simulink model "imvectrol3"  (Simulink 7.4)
settings: Solver=ode23tb  StartTime=0.0  StopTime=1  RelTol=1e-3  AbsTol=1e-3
StartFcn:
  | load('IC3.mat')

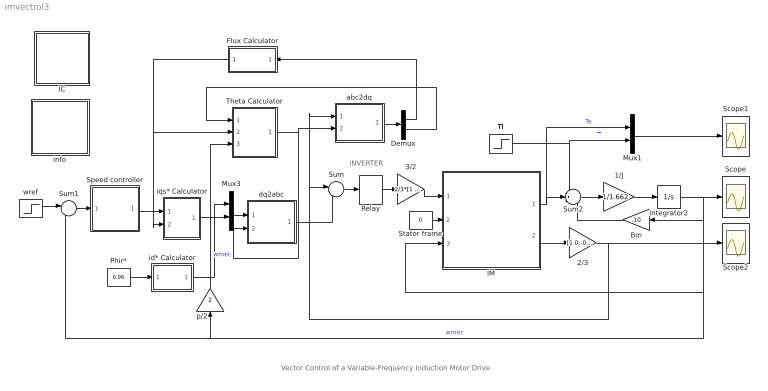
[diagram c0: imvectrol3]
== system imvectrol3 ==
  note: Vector Control of a Variable-Frequency Induction Motor Drive
  note: INVERTER
  1/J : Gain  Gain=1/1.662
  2/3 : Gain  Gain=[1 0;-0.5 sqrt(3)/2;-0.5 -sqrt(3)/2]  Multiplication=Matrix(K*u)
  3/2 : Gain  Gain=2/3*[1 -.5 -.5;0 sqrt(3)/2 -sqrt(3)/2]  Multiplication=Matrix(K*u)
  Bm : Gain  Gain=.10
  Demux : Demux  Outputs=2
  Flux Calculator : Subsystem
  IC : Subsystem
  IM : Subsystem  mask{Rs=0.087, Lsl=0.8e-3, Rr=0.228, Lrl=0.8e-3, Lm=34.7e-3, p=4}
      mask prompts: Rs "Stator resistance [ohm]"; Lsl "Stator leakage inductance [H]"; Rr "Rotor resistance [ohm]"; Lrl "Rotor leakage inductance [H]"; Lm "Magnetizing inductance [H]"; p "Number of poles"
  Integrator2 : Integrator
  Mux1 : Mux  Inputs=2
  Mux3 : Mux  Inputs=2
  Phir* : Constant  Value=0.96
  Relay : Relay  OnSwitchValue=10  OffSwitchValue=-10  OnOutputValue=780  OffOutputValue=-780
  Scope : Scope
  Scope1 : Scope
  Scope2 : Scope
  Speed controller : Subsystem  mask(PI controller){Kp=100, Ki=5200, Tlim=300, Ts=0}
      mask prompts: Kp "Proportional gain (Kp)"; Ki "Integral gain (Ki)"; Tlim "Torque limit (N.m)"; Ts "Sampling time (s)"
      mask help: Proportional-Integral Speed Controller
  Stator frame : Constant  Value=0
  Sum : Sum  Inputs=|-+
  Sum1 : Sum  Inputs=|+-
  Sum2 : Sum  Inputs=-+-
  Theta Calculator : Subsystem
  Tl : Step  Time=0.6  After=200  SampleTime=0
  abc2dq : Subsystem
  dq2abc : Subsystem
  id* Calculator : Subsystem
  info : Subsystem
  iqs* Calculator : Subsystem
  p/2 : Gain  Gain=2
  wref : Step  Time=0.1  Before=120  After=150  SampleTime=0
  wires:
  Phir*/1 -> id* Calculator/1(Phir*)
  iqs* Calculator/1(Iq*) -> Mux3/2
  id* Calculator/1(Id*) -> Mux3/1
  Flux Calculator/1(Phir) -> Theta Calculator/2(Phir), iqs* Calculator/2(Phir)
  wref/1 -> Sum1/1
  Sum2/1 -> 1/J/1
  1/J/1 -> Integrator2/1
  Integrator2/1 -> Bm/1, IM/3(wmec), Sum1/2, p/2/1, Scope/1  "wmec"
  Bm/1 -> Sum2/3
  IM/1(Te) -> Sum2/2, Mux1/1  "Te"
  Stator frame/1 -> IM/2(wk)
  IM/2(is) -> 2/3/1
  2/3/1 -> Scope2/1, Sum/1, abc2dq/1(iabc)
  Sum/1 -> Relay/1
  3/2/1 -> IM/1(vs)
  Relay/1 -> 3/2/1
  Mux3/1 -> dq2abc/1(idq)
  dq2abc/1(iabc^) -> Sum/2
  Theta Calculator/1(theta) -> dq2abc/2(theta), abc2dq/2(theta)
  Demux/1 -> Flux Calculator/1(Id)
  Demux/2 -> Theta Calculator/1(Iq)
  Speed controller/1(Te*) -> iqs* Calculator/1(Te*)
  Sum1/1 -> Speed controller/1(we)
  abc2dq/1(idq) -> Demux/1
  p/2/1 -> Theta Calculator/3(wm)  "wmec"
  Mux1/1 -> Scope1/1
  Tl/1 -> Mux1/2, Sum2/1  "Tl"

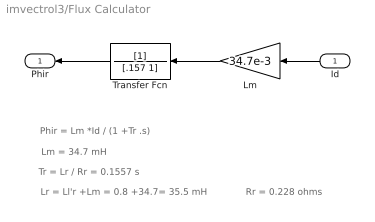
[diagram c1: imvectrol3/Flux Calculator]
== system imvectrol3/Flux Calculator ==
  note: Phir = Lm *Id / (1 +Tr .s)
  note: Lm = 34.7 mH
  note: Lr = Ll'r +Lm = 0.8 +34.7= 35.5 mH
  note: Tr = Lr / Rr = 0.1557 s
  note: Rr = 0.228 ohms
  Id : Inport
  Lm : Gain  Gain=34.7e-3
  Transfer Fcn : TransferFcn  Denominator=[.157 1]
  Phir : Outport
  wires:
  Transfer Fcn/1 -> Phir/1
  Id/1 -> Lm/1
  Lm/1 -> Transfer Fcn/1

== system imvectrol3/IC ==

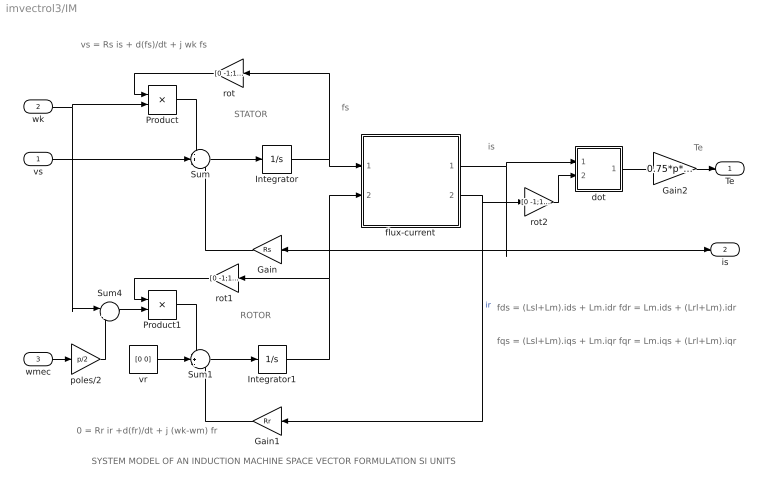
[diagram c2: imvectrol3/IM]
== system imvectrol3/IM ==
  note: fqs = (Lsl+Lm).iqs + Lm.iqr fqr = Lm.iqs + (Lrl+Lm).iqr
  note: fds = (Lsl+Lm).ids + Lm.idr fdr = Lm.ids + (Lrl+Lm).idr
  note: 0 = Rr ir +d(fr)/dt + j (wk-wm) fr
  note: vs = Rs is + d(fs)/dt + j wk fs
  note: SYSTEM MODEL OF AN INDUCTION MACHINE SPACE VECTOR FORMULATION SI UNITS
  note: Te
  note: is
  note: fs
  note: STATOR
  note: ROTOR
  vs : Inport
  wk : Inport  Port=2
  wmec : Inport  Port=3
  Gain : Gain  Gain=Rs
  Gain1 : Gain  Gain=Rr
  Gain2 : Gain  Gain=0.75*p*Lm
  Integrator : Integrator  InitialCondition=[0 0]
  Integrator1 : Integrator  InitialCondition=[0 0]
  Product : Product
  Product1 : Product
  Sum : Sum  Inputs=-+-
  Sum1 : Sum  Inputs=-+-
  Sum4 : Sum  Inputs=|+-
  dot : Subsystem
  flux-current : Subsystem
  poles/2 : Gain  Gain=p/2
  rot : Gain  Gain=[0 -1;1 0]  Multiplication=Matrix(K*u)
  rot1 : Gain  Gain=[0 -1;1 0]  Multiplication=Matrix(K*u)
  rot2 : Gain  Gain=[0 -1;1 0]  Multiplication=Matrix(K*u)
  vr : Constant  Value=[0 0]
  Te : Outport
  is : Outport  Port=2
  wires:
  poles/2/1 -> Sum4/2
  wmec/1 -> poles/2/1
  Gain2/1 -> Te/1
  dot/1(Te) -> Gain2/1
  flux-current/2(ir) -> rot2/1, Gain1/1  "ir"
  flux-current/1(is) -> dot/1(is), is/1, Gain/1
  Sum/1 -> Integrator/1
  Sum1/1 -> Integrator1/1
  wk/1 -> Sum4/1, Product/2
  vs/1 -> Sum/2
  Sum4/1 -> Product1/2
  rot/1 -> Product/1
  Product/1 -> Sum/1
  rot1/1 -> Product1/1
  Product1/1 -> Sum1/1
  Integrator1/1 -> rot1/1, flux-current/2(fr)
  Integrator/1 -> rot/1, flux-current/1(fs)
  Gain1/1 -> Sum1/3
  vr/1 -> Sum1/2
  Gain/1 -> Sum/3
  rot2/1 -> dot/2(jir)

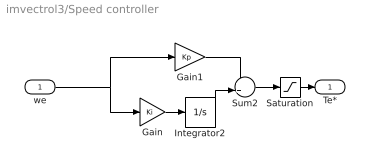
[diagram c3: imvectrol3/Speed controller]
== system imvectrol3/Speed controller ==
  we : Inport
  Gain : Gain  Gain=Ki
  Gain1 : Gain  Gain=Kp
  Integrator2 : Integrator  LimitOutput=on  UpperSaturationLimit=Tlim  LowerSaturationLimit=-Tlim
  Saturation : Saturate  UpperLimit=Tlim  LowerLimit=-Tlim
  Sum2 : Sum
  Te* : Outport  InitialOutput=0
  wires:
  Gain1/1 -> Sum2/1
  Gain/1 -> Integrator2/1
  Saturation/1 -> Te*/1
  we/1 -> Gain/1, Gain1/1
  Sum2/1 -> Saturation/1
  Integrator2/1 -> Sum2/2

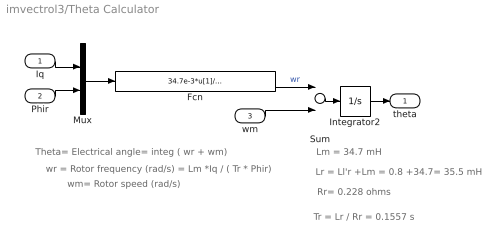
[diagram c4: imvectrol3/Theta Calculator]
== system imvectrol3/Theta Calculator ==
  note: Theta= Electrical angle= integ ( wr + wm)
  note: wr = Rotor frequency (rad/s) = Lm *Iq / ( Tr * Phir)
  note: Lm = 34.7 mH
  note: Rr= 0.228 ohms
  note: Lr = Ll'r +Lm = 0.8 +34.7= 35.5 mH
  note: wm= Rotor speed (rad/s)
  note: Tr = Lr / Rr = 0.1557 s
  Iq : Inport
  Phir : Inport  Port=2
  wm : Inport  Port=3
  Fcn : Fcn  Expr=34.7e-3*u[1]/(u[2]*0.1557+1e-3)
  Integrator2 : Integrator
  Mux : Mux  Inputs=2
  Sum : Sum
  theta : Outport  InitialOutput=0
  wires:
  Integrator2/1 -> theta/1
  Sum/1 -> Integrator2/1
  wm/1 -> Sum/2
  Fcn/1 -> Sum/1  "wr"
  Phir/1 -> Mux/2
  Iq/1 -> Mux/1
  Mux/1 -> Fcn/1

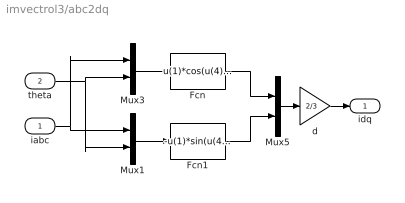
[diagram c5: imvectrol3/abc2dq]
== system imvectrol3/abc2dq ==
  iabc : Inport
  theta : Inport  Port=2
  Fcn : Fcn  Expr=u(1)*cos(u(4))+u(2)*cos(u(4)-2*pi/3)+u(3)*cos(u(4)+2*pi/3)
  Fcn1 : Fcn  Expr=-u(1)*sin(u(4))-u(2)*sin(u(4)-2*pi/3)-u(3)*sin(u(4)+2*pi/3)
  Mux1 : Mux  Inputs=2
  Mux3 : Mux  Inputs=2
  Mux5 : Mux  Inputs=2
  d : Gain  Gain=2/3
  idq : Outport
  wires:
  Mux3/1 -> Fcn/1
  Fcn/1 -> Mux5/1
  Mux5/1 -> d/1
  Mux1/1 -> Fcn1/1
  Fcn1/1 -> Mux5/2
  iabc/1 -> Mux1/1, Mux3/1
  theta/1 -> Mux3/2, Mux1/2
  d/1 -> idq/1

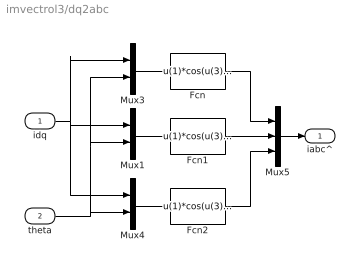
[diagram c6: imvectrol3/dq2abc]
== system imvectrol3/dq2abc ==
  idq : Inport
  theta : Inport  Port=2
  Fcn : Fcn  Expr=u(1)*cos(u(3))-u(2)*sin(u(3))
  Fcn1 : Fcn  Expr=u(1)*cos(u(3)-2*pi/3)-u(2)*sin(u(3)-2*pi/3)
  Fcn2 : Fcn  Expr=u(1)*cos(u(3)+2*pi/3)-u(2)*sin(u(3)+2*pi/3)
  Mux1 : Mux  Inputs=2
  Mux3 : Mux  Inputs=2
  Mux4 : Mux  Inputs=2
  Mux5 : Mux  Inputs=3
  iabc^ : Outport
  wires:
  Mux3/1 -> Fcn/1
  Mux4/1 -> Fcn2/1
  idq/1 -> Mux3/1, Mux4/1, Mux1/1
  Fcn/1 -> Mux5/1
  Mux5/1 -> iabc^/1
  Mux1/1 -> Fcn1/1
  Fcn1/1 -> Mux5/2
  Fcn2/1 -> Mux5/3
  theta/1 -> Mux4/2, Mux3/2, Mux1/2

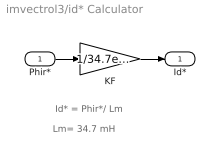
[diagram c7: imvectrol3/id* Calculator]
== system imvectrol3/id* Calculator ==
  note: Id* = Phir*/ Lm
  note: Lm= 34.7 mH
  Phir* : Inport
  KF : Gain  Gain=1/34.7e-3
  Id* : Outport
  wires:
  KF/1 -> Id*/1
  Phir*/1 -> KF/1

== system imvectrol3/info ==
  note: A three-phase induction motor rated at 50hp, 460V,4pole,60Hz is modeled in the common stator reference frame.The speed loop utilizes a PI controller to produce the quadrature-axis currents iq* which serves as the torque command. The derived direct-axis current id* serves as the rotor flux command. These currents are then transformed via the block into the currrent references ia*, ib*, and ic* fed into the current regulator. The current-controlled PWM inverter is made up of three hysteresis controllers. Rotor flux field orientation is obtained in the block. First double-click to establish the specific steady-state operation at wref=120rad/s and Tl=0. Then examine the transient response due to step changes in the command speed wref and load torque Tl. Repeat the simulation for a so-called detuned case when the estimated value of the rotor time constant Tr appearing in the differs from the actual value used for the motor parameters.
  note: (adapted from Power System Blockset case study)
  note: Indirect Vector Control of a Variable-Frequency Induction Motor Drive

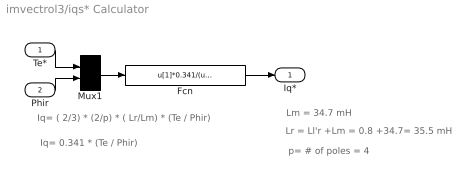
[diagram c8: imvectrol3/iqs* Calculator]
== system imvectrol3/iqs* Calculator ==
  note: Iq= ( 2/3) * (2/p) * ( Lr/Lm) * (Te / Phir)
  note: Lm = 34.7 mH
  note: Lr = Ll'r +Lm = 0.8 +34.7= 35.5 mH
  note: p= # of poles = 4
  note: Iq= 0.341 * (Te / Phir)
  Te* : Inport
  Phir : Inport  Port=2
  Fcn : Fcn  Expr=u[1]*0.341/(u[2]+1e-3)
  Mux1 : Mux  Inputs=2
  Iq* : Outport  InitialOutput=0
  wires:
  Phir/1 -> Mux1/2
  Fcn/1 -> Iq*/1
  Te*/1 -> Mux1/1
  Mux1/1 -> Fcn/1

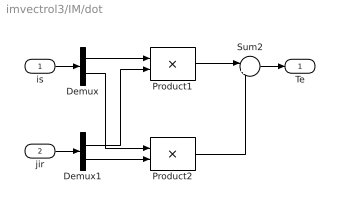
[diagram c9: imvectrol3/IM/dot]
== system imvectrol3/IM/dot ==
  is : Inport
  jir : Inport  Port=2
  Demux : Demux  Outputs=2
  Demux1 : Demux  Outputs=2
  Product1 : Product
  Product2 : Product
  Sum2 : Sum  Inputs=|++
  Te : Outport
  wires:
  Demux/1 -> Product1/1
  Demux1/2 -> Product2/2
  Demux/2 -> Product2/1
  Demux1/1 -> Product1/2
  Product1/1 -> Sum2/1
  Product2/1 -> Sum2/2
  Sum2/1 -> Te/1
  is/1 -> Demux/1
  jir/1 -> Demux1/1

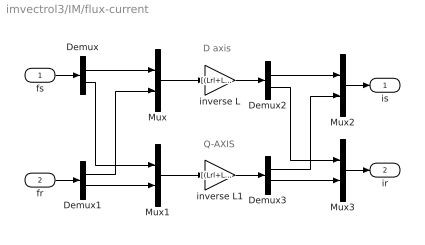
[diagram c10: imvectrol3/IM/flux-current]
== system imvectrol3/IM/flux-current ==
  note: Q-AXIS
  note: D axis
  fs : Inport
  fr : Inport  Port=2
  Demux{,1..3} (4 alike) : Demux  Outputs=2
  Mux{,1..3} (4 alike) : Mux  Inputs=2
  inverse L : Gain  Gain=[(Lrl+Lm) -Lm;-Lm (Lsl+Lm)]/(Lsl*Lrl+Lsl*Lm+Lrl*Lm)  Multiplication=Matrix(K*u)
  inverse L1 : Gain  Gain=[(Lrl+Lm) -Lm;-Lm (Lsl+Lm)]/(Lsl*Lrl+Lsl*Lm+Lrl*Lm)  Multiplication=Matrix(K*u)
  is : Outport
  ir : Outport  Port=2
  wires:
  fr/1 -> Demux1/1
  Mux3/1 -> ir/1
  Demux3/1 -> Mux2/2
  Demux2/2 -> Mux3/1
  Demux3/2 -> Mux3/2
  inverse L1/1 -> Demux3/1
  Mux1/1 -> inverse L1/1
  Demux/2 -> Mux1/1
  Demux1/2 -> Mux1/2
  Demux1/1 -> Mux/2
  Mux2/1 -> is/1
  fs/1 -> Demux/1
  Demux2/1 -> Mux2/1
  inverse L/1 -> Demux2/1
  Mux/1 -> inverse L/1
  Demux/1 -> Mux/1
